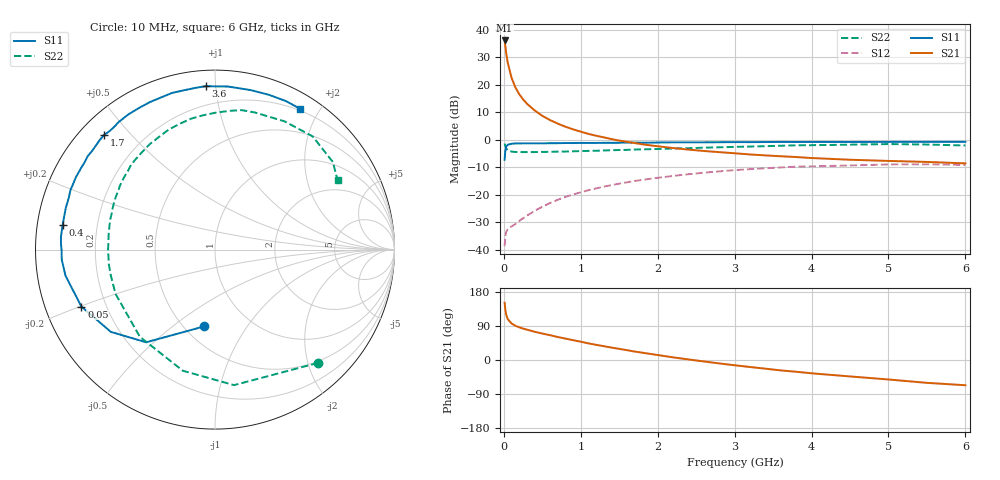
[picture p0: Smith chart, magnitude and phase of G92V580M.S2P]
! SIEMENS Small Signal Semiconductors
! BFG235
! Si NPN RF Bipolar Junction Transistor in SOT223
! VCE = 2.5 V  IC = 80 mA
! Common Emitter S-Parameters:  July  1994
# GHz  S  MA  R  50
!  f  S11  S21  S12  S22
! GHz  MAG  ANG  MAG  ANG  MAG  ANG  MAG  ANG
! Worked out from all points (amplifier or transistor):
!   40 points, 10 MHz to 6 GHz, reference 50 ohm
!   highest |S21| = 36.2 dB at 10 MHz (marker M1)
!   |S21| within 3 dB of that: start of sweep to 23.43 MHz
!   unconditionally stable (mu >= 1): 466.2 MHz to 1.525 GHz
!   at 200 MHz: K = 0.76, MSG = 23.1 dB, |S12| = -29.6 dB
!   at 1.5 GHz: K = 1.00, MAG = 7.4 dB, |S12| = -16.0 dB
!   at 6 GHz: K = 0.92, MSG = 0.3 dB, |S12| = -9.2 dB
!   S11 on the Smith chart (normalised r, x): 10 MHz: 0.62, -0.66; 50 MHz: 0.11, -0.20; 400 MHz: 0.08, +0.08; 1.7 GHz: 0.07, +0.42; 3.6 GHz: 0.09, +0.94; 6 GHz: 0.18, +1.76
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0.01  0.4317 -97.9  64.37 151.2  0.0115 62.6  0.8532 -47.7
0.02  0.6433 -126.6  49.69 132.1  0.0174 46.9  0.7625 -82.0
0.03  0.7396 -141.7  38.6 120.3  0.0208 38.2  0.6983 -104.9
0.05  0.8092 -156.9  25.51 108.1  0.0233 31.5  0.6412 -130.8
0.1  0.8455 -170.1  13.42 96.3  0.0263 32.4  0.6067 -156.0
0.15  0.8556 -176.2  9.003 90.3  0.0291 38.2  0.598 -166.3
0.2  0.8544 -179.5  6.735 86.3  0.0332 42.6  0.5969 -172.1
0.25  0.8589 177.7  5.43 82.9  0.0371 46.2  0.5949 -176.2
0.3  0.8613 175.2  4.536 80.1  0.0413 49.4  0.5959 -179.6
0.4  0.86 170.9  3.416 74.6  0.0505 52.6  0.5956 175.5
0.5  0.8605 167.3  2.726 69.8  0.0602 54.4  0.5992 171.3
0.6  0.8633 164.3  2.281 65.5  0.0702 54.8  0.6024 167.6
0.7  0.8641 160.6  1.968 60.7  0.0805 54.8  0.6072 164.1
0.9  0.8711 155.0  1.547 52.3  0.1004 52.6  0.6152 157.9
1.1  0.8737 148.6  1.276 43.8  0.1204 49.6  0.6263 151.9
1.7  0.8884 133.9  0.87 22.3  0.177 37.9  0.6625 135.4
2.2  0.8946 122.6  0.705 7.0  0.2191 26.9  0.6911 121.6
3.2  0.9043 101.1  0.539 -18.5  0.291 3.7  0.7508 95.3
3.6  0.9123 93.1  0.5 -27.5  0.313 -6.2  0.7768 84.2
4.5  0.9106 77.4  0.432 -43.4  0.34 -25.9  0.8129 61.5
5.5  0.917 64.5  0.394 -60.3  0.3573 -47.5  0.8181 36.6
6  0.9169 58.7  0.371 -66.6  0.3469 -55.7  0.7844 29.4
